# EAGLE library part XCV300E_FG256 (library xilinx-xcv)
xcv300e_fg256 edit this description Auto generated by make-symbol-device-package-bsdl.ulp Rev. 26 Source: xcv300e_fg256.bsd
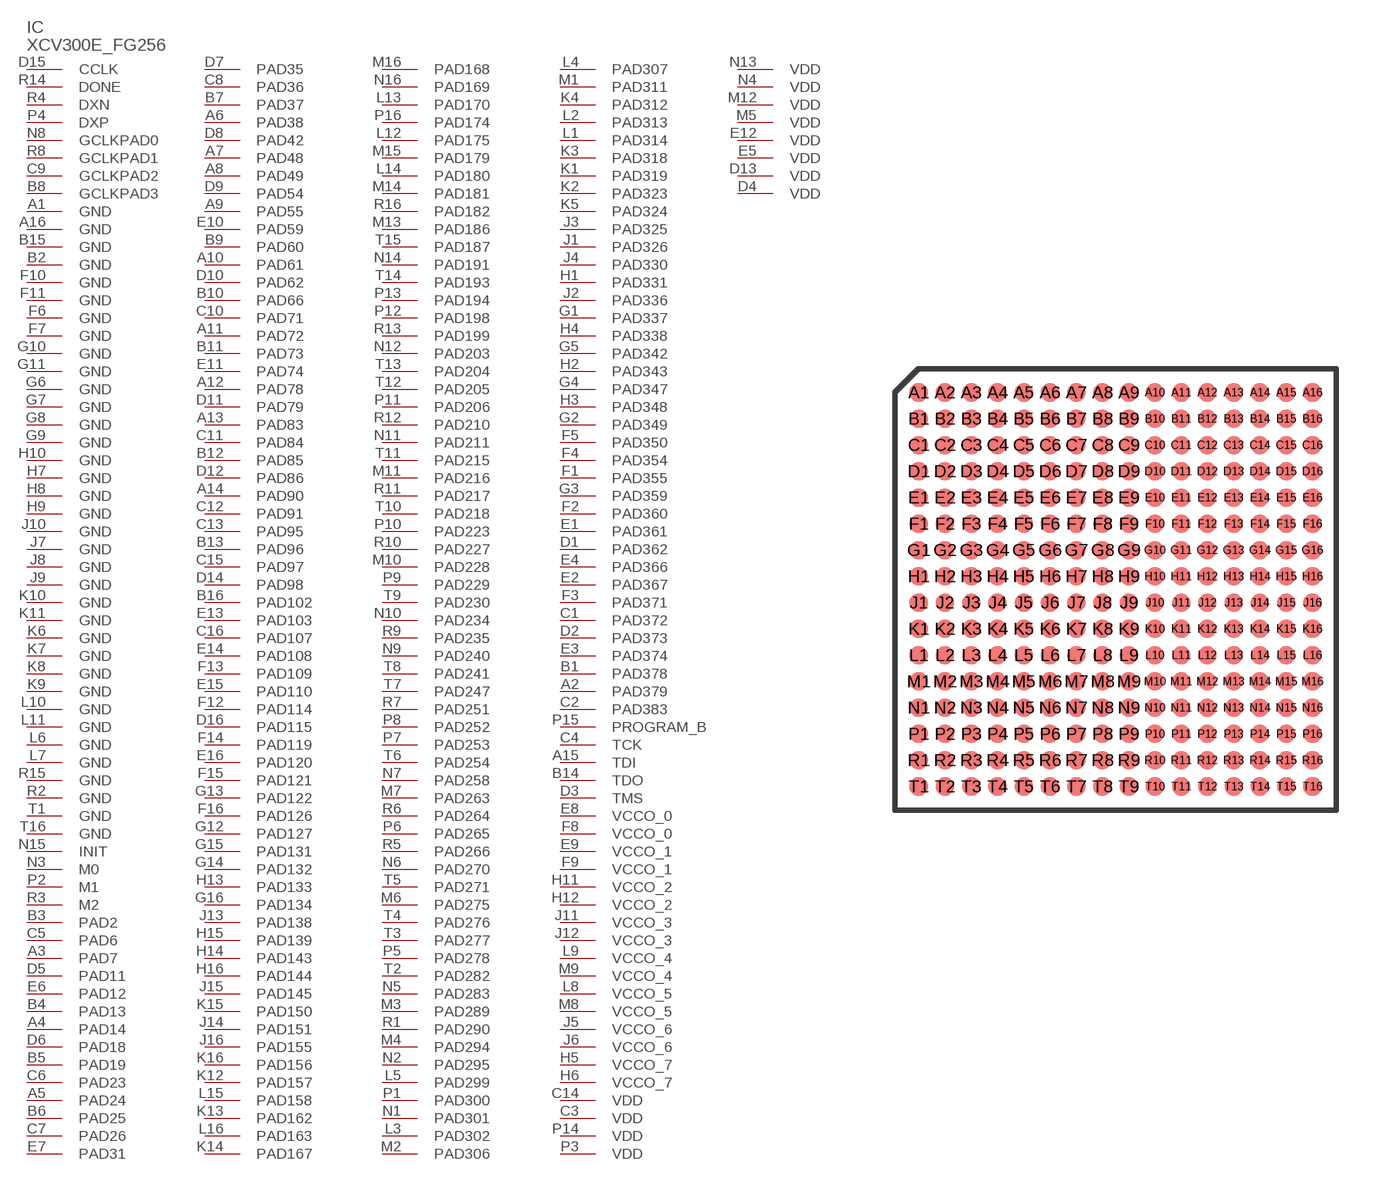
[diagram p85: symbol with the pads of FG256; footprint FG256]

Designator prefix IC

## XCV300E_FG256 (OC_FARNELL: unknown; OC_NEWARK: unknown)  [FG256]
A1  GND  pwr
A2  PAD379
A3  PAD7
A4  PAD14
A5  PAD24
A6  PAD38
A7  PAD48
A8  PAD49
A9  PAD55
A10  PAD61
A11  PAD72
A12  PAD78
A13  PAD83
A14  PAD90
A15  TDI  in
A16  GND  pwr
B1  PAD378
B2  GND  pwr
B3  PAD2
B4  PAD13
B5  PAD19
B6  PAD25
B7  PAD37
B8  GCLKPAD3  in
B9  PAD60
B10  PAD66
B11  PAD73
B12  PAD85
B13  PAD96
B14  TDO  out
B15  GND  pwr
B16  PAD102
C1  PAD372
C2  PAD383
C3  VDD  pwr
C4  TCK  in
C5  PAD6
C6  PAD23
C7  PAD26
C8  PAD36
C9  GCLKPAD2  in
C10  PAD71
C11  PAD84
C12  PAD91
C13  PAD95
C14  VDD  pwr
C15  PAD97
C16  PAD107
D1  PAD362
D2  PAD373
D3  TMS  in
D4  VDD  pwr
D5  PAD11
D6  PAD18
D7  PAD35
D8  PAD42
D9  PAD54
D10  PAD62
D11  PAD79
D12  PAD86
D13  VDD  pwr
D14  PAD98
D15  CCLK
D16  PAD115
E1  PAD361
E2  PAD367
E3  PAD374
E4  PAD366
E5  VDD  pwr
E6  PAD12
E7  PAD31
E8  VCCO_0  pwr
E9  VCCO_1  pwr
E10  PAD59
E11  PAD74
E12  VDD  pwr
E13  PAD103
E14  PAD108
E15  PAD110
E16  PAD120
F1  PAD355
F2  PAD360
F3  PAD371
F4  PAD354
F5  PAD350
F6  GND  pwr
F7  GND  pwr
F8  VCCO_0  pwr
F9  VCCO_1  pwr
F10  GND  pwr
F11  GND  pwr
F12  PAD114
F13  PAD109
F14  PAD119
F15  PAD121
F16  PAD126
G1  PAD337
G2  PAD349
G3  PAD359
G4  PAD347
G5  PAD342
G6  GND  pwr
G7  GND  pwr
G8  GND  pwr
G9  GND  pwr
G10  GND  pwr
G11  GND  pwr
G12  PAD127
G13  PAD122
G14  PAD132
G15  PAD131
G16  PAD134
H1  PAD331
H2  PAD343
H3  PAD348
H4  PAD338
H5  VCCO_7  pwr
H6  VCCO_7  pwr
H7  GND  pwr
H8  GND  pwr
H9  GND  pwr
H10  GND  pwr
H11  VCCO_2  pwr
H12  VCCO_2  pwr
H13  PAD133
H14  PAD143
H15  PAD139
H16  PAD144
J1  PAD326
J2  PAD336
J3  PAD325
J4  PAD330
J5  VCCO_6  pwr
J6  VCCO_6  pwr
J7  GND  pwr
J8  GND  pwr
J9  GND  pwr
J10  GND  pwr
J11  VCCO_3  pwr
J12  VCCO_3  pwr
J13  PAD138
J14  PAD151
J15  PAD145
J16  PAD155
K1  PAD319
K2  PAD323
K3  PAD318
K4  PAD312
K5  PAD324
K6  GND  pwr
K7  GND  pwr
K8  GND  pwr
K9  GND  pwr
K10  GND  pwr
K11  GND  pwr
K12  PAD157
K13  PAD162
K14  PAD167
K15  PAD150
K16  PAD156
L1  PAD314
L2  PAD313
L3  PAD302
L4  PAD307
L5  PAD299
L6  GND  pwr
L7  GND  pwr
L8  VCCO_5  pwr
L9  VCCO_4  pwr
L10  GND  pwr
L11  GND  pwr
L12  PAD175
L13  PAD170
L14  PAD180
L15  PAD158
L16  PAD163
M1  PAD311
M2  PAD306
M3  PAD289
M4  PAD294
M5  VDD  pwr
M6  PAD275
M7  PAD263
M8  VCCO_5  pwr
M9  VCCO_4  pwr
M10  PAD228
M11  PAD216
M12  VDD  pwr
M13  PAD186
M14  PAD181
M15  PAD179
M16  PAD168
N1  PAD301
N2  PAD295
N3  M0  in
N4  VDD  pwr
N5  PAD283
N6  PAD270
N7  PAD258
N8  GCLKPAD0  in
N9  PAD240
N10  PAD234
N11  PAD211
N12  PAD203
N13  VDD  pwr
N14  PAD191
N15  INIT
N16  PAD169
P1  PAD300
P2  M1  in
P3  VDD  pwr
P4  DXP  pas
P5  PAD278
P6  PAD265
P7  PAD253
P8  PAD252
P9  PAD229
P10  PAD223
P11  PAD206
P12  PAD198
P13  PAD194
P14  VDD  pwr
P15  PROGRAM_B  in
P16  PAD174
R1  PAD290
R2  GND  pwr
R3  M2  in
R4  DXN  pas
R5  PAD266
R6  PAD264
R7  PAD251
R8  GCLKPAD1  in
R9  PAD235
R10  PAD227
R11  PAD217
R12  PAD210
R13  PAD199
R14  DONE
R15  GND  pwr
R16  PAD182
T1  GND  pwr
T2  PAD282
T3  PAD277
T4  PAD276
T5  PAD271
T6  PAD254
T7  PAD247
T8  PAD241
T9  PAD230
T10  PAD218
T11  PAD215
T12  PAD205
T13  PAD204
T14  PAD193
T15  PAD187
T16  GND  pwr

## Footprint FG256 (pad centres in mm)
Fine Pitch BGA (FG256) Auto generated by make-symbol-device-package-bsdl.ulp Rev. 26 Source: xcv100_fg256.bsd; fg256.pdf
smd 0.7 x 0.7: A1 -7.5,7.5; A2 -6.5,7.5; A3 -5.5,7.5; A4 -4.5,7.5; A5 -3.5,7.5; A6 -2.5,7.5; A7 -1.5,7.5; A8 -0.5,7.5; A9 0.5,7.5; A10 1.5,7.5; A11 2.5,7.5; A12 3.5,7.5; A13 4.5,7.5; A14 5.5,7.5; A15 6.5,7.5; A16 7.5,7.5; B1 -7.5,6.5; B2 -6.5,6.5; B3 -5.5,6.5; B4 -4.5,6.5; B5 -3.5,6.5; B6 -2.5,6.5; B7 -1.5,6.5; B8 -0.5,6.5; B9 0.5,6.5; B10 1.5,6.5; B11 2.5,6.5; B12 3.5,6.5; B13 4.5,6.5; B14 5.5,6.5; B15 6.5,6.5; B16 7.5,6.5; C1 -7.5,5.5; C2 -6.5,5.5; C3 -5.5,5.5; C4 -4.5,5.5; C5 -3.5,5.5; C6 -2.5,5.5; C7 -1.5,5.5; C8 -0.5,5.5; C9 0.5,5.5; C10 1.5,5.5; C11 2.5,5.5; C12 3.5,5.5; C13 4.5,5.5; C14 5.5,5.5; C15 6.5,5.5; C16 7.5,5.5; D1 -7.5,4.5; D2 -6.5,4.5; D3 -5.5,4.5; D4 -4.5,4.5; D5 -3.5,4.5; D6 -2.5,4.5; D7 -1.5,4.5; D8 -0.5,4.5; D9 0.5,4.5; D10 1.5,4.5; D11 2.5,4.5; D12 3.5,4.5; D13 4.5,4.5; D14 5.5,4.5; D15 6.5,4.5; D16 7.5,4.5; E1 -7.5,3.5; E2 -6.5,3.5; E3 -5.5,3.5; E4 -4.5,3.5; E5 -3.5,3.5; E6 -2.5,3.5; E7 -1.5,3.5; E8 -0.5,3.5; E9 0.5,3.5; E10 1.5,3.5; E11 2.5,3.5; E12 3.5,3.5; E13 4.5,3.5; E14 5.5,3.5; E15 6.5,3.5; E16 7.5,3.5; F1 -7.5,2.5; F2 -6.5,2.5; F3 -5.5,2.5; F4 -4.5,2.5; F5 -3.5,2.5; F6 -2.5,2.5; F7 -1.5,2.5; F8 -0.5,2.5; F9 0.5,2.5; F10 1.5,2.5; F11 2.5,2.5; F12 3.5,2.5; F13 4.5,2.5; F14 5.5,2.5; F15 6.5,2.5; F16 7.5,2.5; G1 -7.5,1.5; G2 -6.5,1.5; G3 -5.5,1.5; G4 -4.5,1.5; G5 -3.5,1.5; G6 -2.5,1.5; G7 -1.5,1.5; G8 -0.5,1.5; G9 0.5,1.5; G10 1.5,1.5; G11 2.5,1.5; G12 3.5,1.5; G13 4.5,1.5; G14 5.5,1.5; G15 6.5,1.5; G16 7.5,1.5; H1 -7.5,0.5; H2 -6.5,0.5; H3 -5.5,0.5; H4 -4.5,0.5; H5 -3.5,0.5; H6 -2.5,0.5; H7 -1.5,0.5; H8 -0.5,0.5; H9 0.5,0.5; H10 1.5,0.5; H11 2.5,0.5; H12 3.5,0.5; H13 4.5,0.5; H14 5.5,0.5; H15 6.5,0.5; H16 7.5,0.5; J1 -7.5,-0.5; J2 -6.5,-0.5; J3 -5.5,-0.5; J4 -4.5,-0.5; J5 -3.5,-0.5; J6 -2.5,-0.5; J7 -1.5,-0.5; J8 -0.5,-0.5; J9 0.5,-0.5; J10 1.5,-0.5; J11 2.5,-0.5; J12 3.5,-0.5; J13 4.5,-0.5; J14 5.5,-0.5; J15 6.5,-0.5; J16 7.5,-0.5; K1 -7.5,-1.5; K2 -6.5,-1.5; K3 -5.5,-1.5; K4 -4.5,-1.5; K5 -3.5,-1.5; K6 -2.5,-1.5; K7 -1.5,-1.5; K8 -0.5,-1.5; K9 0.5,-1.5; K10 1.5,-1.5; K11 2.5,-1.5; K12 3.5,-1.5; K13 4.5,-1.5; K14 5.5,-1.5; K15 6.5,-1.5; K16 7.5,-1.5; L1 -7.5,-2.5; L2 -6.5,-2.5; L3 -5.5,-2.5; L4 -4.5,-2.5; L5 -3.5,-2.5; L6 -2.5,-2.5; L7 -1.5,-2.5; L8 -0.5,-2.5; L9 0.5,-2.5; L10 1.5,-2.5; L11 2.5,-2.5; L12 3.5,-2.5; L13 4.5,-2.5; L14 5.5,-2.5; L15 6.5,-2.5; L16 7.5,-2.5; M1 -7.5,-3.5; M2 -6.5,-3.5; M3 -5.5,-3.5; M4 -4.5,-3.5; M5 -3.5,-3.5; M6 -2.5,-3.5; M7 -1.5,-3.5; M8 -0.5,-3.5; M9 0.5,-3.5; M10 1.5,-3.5; M11 2.5,-3.5; M12 3.5,-3.5; M13 4.5,-3.5; M14 5.5,-3.5; M15 6.5,-3.5; M16 7.5,-3.5; N1 -7.5,-4.5; N2 -6.5,-4.5; N3 -5.5,-4.5; N4 -4.5,-4.5; N5 -3.5,-4.5; N6 -2.5,-4.5; N7 -1.5,-4.5; N8 -0.5,-4.5; N9 0.5,-4.5; N10 1.5,-4.5; N11 2.5,-4.5; N12 3.5,-4.5; N13 4.5,-4.5; N14 5.5,-4.5; N15 6.5,-4.5; N16 7.5,-4.5; P1 -7.5,-5.5; P2 -6.5,-5.5; P3 -5.5,-5.5; P4 -4.5,-5.5; P5 -3.5,-5.5; P6 -2.5,-5.5; P7 -1.5,-5.5; P8 -0.5,-5.5; P9 0.5,-5.5; P10 1.5,-5.5; P11 2.5,-5.5; P12 3.5,-5.5; P13 4.5,-5.5; P14 5.5,-5.5; P15 6.5,-5.5; P16 7.5,-5.5; R1 -7.5,-6.5; R2 -6.5,-6.5; R3 -5.5,-6.5; R4 -4.5,-6.5; R5 -3.5,-6.5; R6 -2.5,-6.5; R7 -1.5,-6.5; R8 -0.5,-6.5; R9 0.5,-6.5; R10 1.5,-6.5; R11 2.5,-6.5; R12 3.5,-6.5; R13 4.5,-6.5; R14 5.5,-6.5; R15 6.5,-6.5; R16 7.5,-6.5; T1 -7.5,-7.5; T2 -6.5,-7.5; T3 -5.5,-7.5; T4 -4.5,-7.5; T5 -3.5,-7.5; T6 -2.5,-7.5; T7 -1.5,-7.5; T8 -0.5,-7.5; T9 0.5,-7.5; T10 1.5,-7.5; T11 2.5,-7.5; T12 3.5,-7.5; T13 4.5,-7.5; T14 5.5,-7.5; T15 6.5,-7.5; T16 7.5,-7.5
